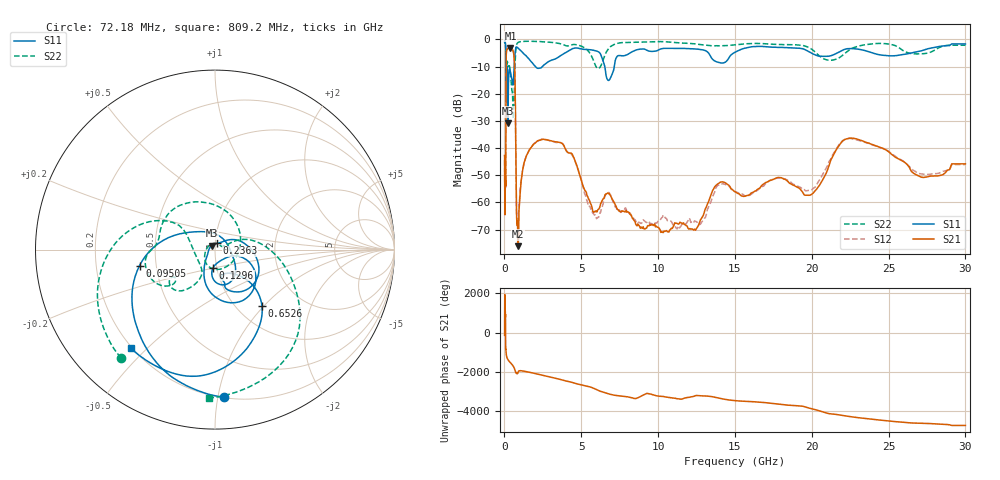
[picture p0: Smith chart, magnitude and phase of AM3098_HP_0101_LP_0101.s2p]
! Date/Time: Thu, Feb 28, 2019 8:36 AM
! Network Analyzer: Agilent Technologies E8364B Rev: A.07.50.67
! Sweep from 0.010 to 30.000 GHz, 1601 Points, Sweep Type: LOG
! Power Supply: 5.022 V, 0.002 A
# Hz S DB R 50
!freq MagS11 AngS11 MagS21 AngS21 MagS12 AngS12 MagS22 AngS22
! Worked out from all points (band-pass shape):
!   1601 points, 10 MHz to 30 GHz, reference 50 ohm
!   highest |S21| = -3.08 dB at 391.7 MHz (marker M1); lowest = -76.1 dB at 881.1 MHz (marker M2)
!   |S21| within 3 dB of the highest: 113.4 MHz to 618.9 MHz (505.5 MHz wide, 138 % of centre)
!   lowest |S11| = -30.8 dB at 229.3 MHz (marker M3), VSWR 1.06, Z = 48.1 + j2.06 ohm
!   |S11| at or under -10 dB: 176.4 MHz to 632.2 MHz (455.8 MHz wide, 113 % of centre); 2.023 GHz to 2.46 GHz (437.5 MHz wide, 19.5 % of centre); 6.528 GHz to 7.147 GHz (618.3 MHz wide, 9.04 % of centre)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
!   |S22| runs from -29.2 to -0.5 dB; largest |S21 - S12| = 0.01
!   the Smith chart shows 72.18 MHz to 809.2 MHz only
!   S11 on the Smith chart (normalised r, x): 72.18 MHz: 0.20, -1.04; 95.05 MHz: 0.40, -0.09; 129.6 MHz: 0.96, -0.19; 236.3 MHz: 1.02, +0.07; 652.6 MHz: 1.29, -0.98; 809.2 MHz: 0.19, -0.45
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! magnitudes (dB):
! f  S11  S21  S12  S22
! 10 MHz  -0.4  -42.7  -44.3  -0.5
! 38.04 MHz  -0.5  -61.6  -59.2  -0.9
! 72.18 MHz  -1.7  -52.2  -53.7  -1.9
! 82.62 MHz  -2.7  -48.9  -51.2  -2.9
! 95.05 MHz  -7.3  -22.5  -22.4  -8.6
! 129.6 MHz  -19.9  -4.5  -4.5  -10.6
! 144.7 MHz  -16.5  -3.8  -3.8  -10.9
! 184.9 MHz  -10.9  -3.6  -3.6  -8.0
! 229.3 MHz  -30.8  -3.2  -3.1  -9.6
! 236.3 MHz  -28.7  -3.2  -3.1  -9.7
! 391.7 MHz  -12.1  -3.1  -3.1  -12.5
! 550.5 MHz  -16.8  -4.1  -4.1  -24.8
! 652.6 MHz  -7.8  -8.7  -8.7  -17.5
! 809.2 MHz  -2.8  -66.6  -66.5  -1.6
! 881.1 MHz  -3.2  -76.1  -66.8  -1.1
! 1.184 GHz  -4.8  -48.2  -48.1  -0.7
! 2.084 GHz  -10.4  -37.7  -37.7  -0.7
! 7.926 GHz  -5.8  -63.0  -62.6  -1.1
! 12.25 GHz  -3.4  -69.9  -67.2  -1.5
! 20 GHz  -5.1  -57.0  -55.3  -3.6
! 22.67 GHz  -3.4  -36.3  -36.7  -3.2
! 30 GHz  -1.6  -45.8  -46.1  -2.1
